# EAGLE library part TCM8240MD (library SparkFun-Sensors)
Toshiba TCM8240MD 1.3MP Color Image Sensor The TCM8240MD is a high quality, very small 1.3 mega-pixel color camera from Toshiba with the standard data+I2C interface. The nice thing is that we have a good supplier of these cameras, so they should be around for some time. This camera is also unique in that it offers on-board JPEG compression. Datasheet SparkFun Products CMOS Camera - 1300x1040 (SEN-08668) TCM8240 Camera Breakout (BOB-09504)
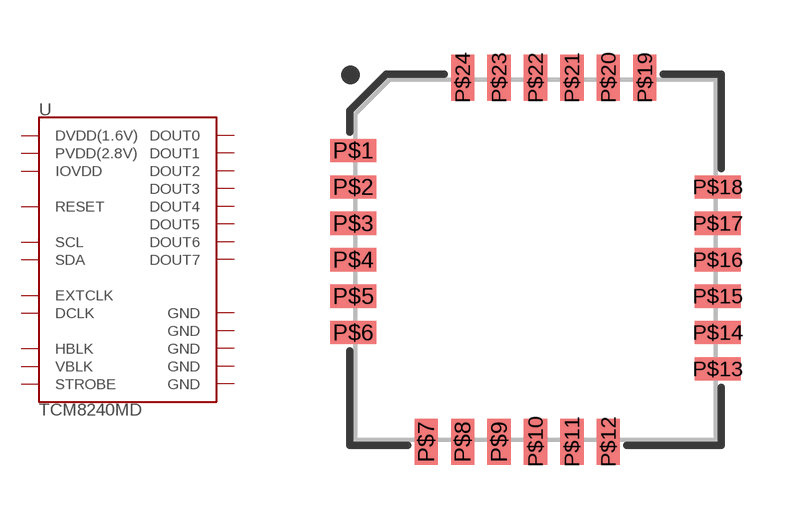
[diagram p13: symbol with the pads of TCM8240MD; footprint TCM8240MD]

Designator prefix U

## TCM8240MD (PROD_ID: COMP-09354; SF_ID: SEN-08668)  [TCM8240MD]
P$1  DOUT3
P$2  DOUT2
P$3  DOUT1
P$4  DOUT0
P$5  GND
P$6  PVDD(2.8V)
P$7  RESET
P$8  SCL
P$9  GND
P$10  SDA
P$11  GND
P$12  DVDD(1.6V)
P$13  EXTCLK
P$14  STROBE
P$15  HBLK
P$16  VBLK
P$17  GND
P$18  IOVDD
P$19  DCLK
P$20  GND
P$21  DOUT7
P$22  DOUT6
P$23  DOUT5
P$24  DOUT4

## Footprint TCM8240MD (pad centres in mm)
TCM8240 CMOS Camera Datasheet Specifications: Pin Count: 24 Area: 10 x 10 x 7.0 mm Pitch: 1 mm Devices Using: TCM8240MD
smd 1.27 x 0.635: P$1 -5,3; P$2 -5,2; P$3 -5,1; P$4 -5,0; P$5 -5,-1; P$6 -5,-2; P$13 5,-3; P$14 5,-2; P$15 5,-1; P$16 5,0; P$17 5,1; P$18 5,2
smd 0.635 x 1.27: P$7 -3,-5; P$8 -2,-5; P$9 -1,-5; P$10 0,-5; P$11 1,-5; P$12 2,-5; P$19 3,5; P$20 2,5; P$21 1,5; P$22 0,5; P$23 -1,5; P$24 -2,5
